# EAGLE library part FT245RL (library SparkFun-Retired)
USB FIFO Controller 4th Generation USB Controller (USB <-> Parallel) - FIFO. Spark Fun Electronics SKU : COM-00787 TODO: Move this to retired
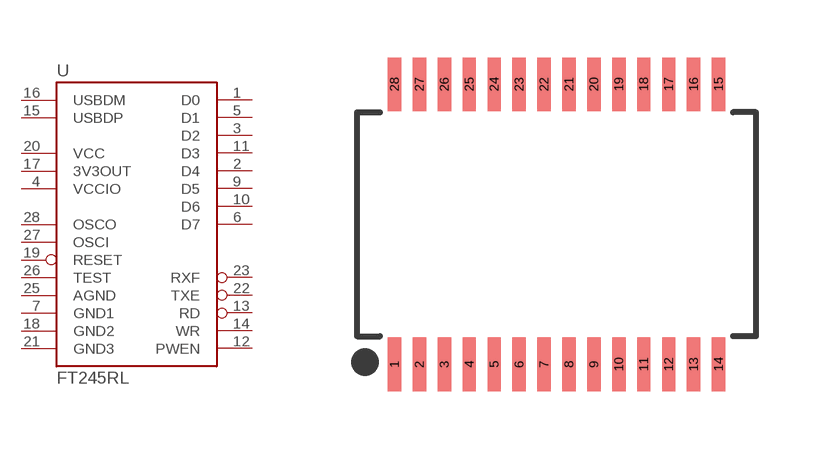
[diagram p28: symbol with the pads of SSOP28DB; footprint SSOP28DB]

Designator prefix -

## FT245RL (PROD_ID: COM-00787; VALUE: FT245RL)  [SSOP28DB]
1  D0  out
2  D4  out
3  D2  out
4  VCCIO  pwr
5  D1  in
6  D7  in
7  GND1  pwr
9  D5  in
10  D6  in
11  D3  in
12  PWEN
13  RD
14  WR
15  USBDP
16  USBDM
17  3V3OUT  out
18  GND2  pwr
19  RESET  in
20  VCC  pwr
21  GND3  pwr
22  TXE
23  RXF
25  AGND  pwr
26  TEST  in
27  OSCI  in
28  OSCO  out

## Footprint SSOP28DB (pad centres in mm)
Small Shrink Outline Package
smd 0.348 x 1.397: 1 -4.225,-3.656; 2 -3.575,-3.656; 3 -2.925,-3.656; 4 -2.275,-3.656; 5 -1.625,-3.656; 6 -0.975,-3.656; 7 -0.325,-3.656; 8 0.325,-3.656; 9 0.975,-3.656; 10 1.625,-3.656; 11 2.275,-3.656; 12 2.925,-3.656; 13 3.575,-3.656; 14 4.225,-3.656; 15 4.225,3.656; 16 3.575,3.656; 17 2.925,3.656; 18 2.275,3.656; 19 1.625,3.656; 20 0.975,3.656; 21 0.325,3.656; 22 -0.325,3.656; 23 -0.975,3.656; 24 -1.625,3.656; 25 -2.275,3.656; 26 -2.925,3.656; 27 -3.575,3.656; 28 -4.225,3.656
